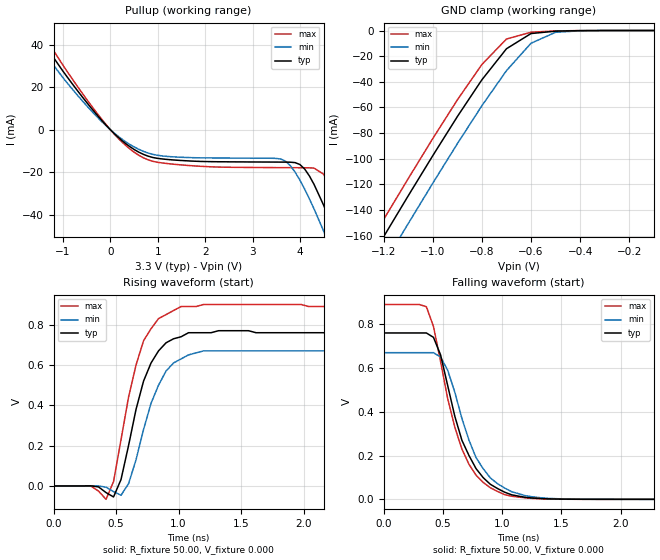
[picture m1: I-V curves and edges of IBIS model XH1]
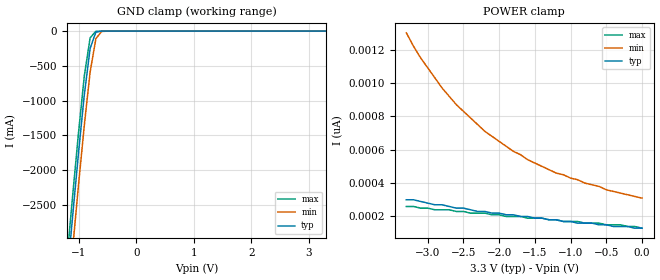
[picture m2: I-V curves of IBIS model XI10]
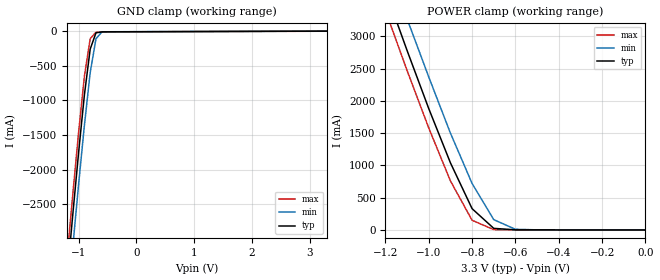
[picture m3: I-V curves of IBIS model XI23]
|   * 9db433a.ibs * IBIS 2.1 Model file
| Rev History
| Rev No.   Description
| 1.0   Initial release   June 6, 2010  lp
[IBIS Ver]   2.1
[Comment char]  |_char
[File name]   9db436a.ibs
[Date]   March 21, 2019
[File Rev]   1.1
[Source]   Originated at Integrated Circuit Systems, Inc.
[Disclaimer] (C) Copyright Integrated Circuit Systems, Inc. 2004
   All rights reserved
ICS hereby grants the user of this IBIS model a non-exclusive,
nontransferable license to use this IBIS model under the following terms.
Before using this IBIS model, the user should read this license.
If the user does not accept these terms,  the IBIS model should be
returned to ICS within 30 days.
   The user is granted this license only to use the IBIS model and
is not granted rights to sell, load, rent, lease or license the IBIS
model in whole or in part, or in modified form to anyone other than
user. User may modify the IBIS model to suit its specific
applications but rights to derivative works and such modifications
shall belong to ICS.
   This IBIS model is provided on an "AS IS" basis and ICS makes
absolutely no warranty with respect to the information contained
herein. ICS DISCLAIMS AND CUSTOMER WAIVES ALL WARRANTIES, EXPRESS
OR IMPLIED, INCLUDING WARRANTIES OF MERCHANTABILITY OR FITNESS FOR
A PARTICULAR PURPOSE. The entire risk as to quality and performance
is with the Customer. ACCORDINGLY, IN NO EVENT SHALL THE COMPANY BE
LIABLE FOR ANY DAMAGES, WHETHER IN CONTRACT OR TORT,INCLUDING ANY
LOST PROFITS OR OTHER INCIDENTAL, CONSEQUENTIAL, EXEMPLARY, OR
PUNITIVE DAMAGES ARISING OUT OF THE USE OR APPLICATION OF THE IBIS
model provided in this package. Further, ICS reserves the right to
make changes without notice to any product herein to improve
reliability, function, or design. ICS does not convey any license
under patent rights or any other intellectual property rights,
including those of third parties.
   ICS is not obligated to provide maintenance or support
for the licensed IBIS model.
|   COMPONENT: ICS9db436a
[Component]   ICS9db436a
[Manufacturer]  ICS
[Package]
| variable   typ   min   max
R_pkg   81.1m   62.2m   100.0m
L_pkg   6.7nH   4.9nH   8.5nH
C_pkg   0.53pF  0.21pF  0.85pF
[Pin]   signal_name   model_name   R_pin   L_pin   C_pin
  1   VDD   POWER   90.5m   4.72nH  0.585pF
  2   SRC_IN   XI4   91.3m   4.11nH  0.57pF
  3   SRC_IN#   XI4   93.6m   3.68nH  0.433pF
  4   GND   GND   39.9m   2.61nH  0.44pF
  5   VDD   POWER   92.1m   3.14nH  0.318pF
  6   DIF_1   XH1   78m   2.79nH  0.286pF
  7   DIF_1#   XH1   70.5m   2.62nH  0.272pF
  8   OE_1(OE_1#)   XI23   39.8m   2.27nH  0.311pF
  9   DIF_2   XH1   74.7m   2.7nH   0.279pF
 10   DIF_2#   XH1   86m   3nH   0.294pF
 11   VDD   POWER   53.2m   2.8nH   0.356pF
 12   BYPASS#/BW   XI23   97.1m   3.84nH  0.432pF
 13   SCLK   XI10   93.6m   4.23nH  0.58pF
 14   SDATA   XIO3   91.4m   4.77nH  0.595pF
 15   GND   GND   91.2m   4.76nH  0.592pF
 16   VDD   POWER   93.7m   4.22nH  0.579pF
 17   SMB_ADR   XI23   97.8m   3.84nH  0.434pF
 18   VDD   POWER   95.6m   3.34nH  0.295pF
 19   DIF_5#   XH1   82.6m   2.93nH  0.285pF
 20   DIF_5   XH1   73.4m   2.67nH  0.277pF
 21   OE_6(OE_6#)   XI23   40m   2.26nH  0.308pF
 22   DIF_6#   XH1   70.8m   2.62nH  0.273pF
 23   DIF_6   XH1   80.8m   2.86nH  0.293pF
 24   VDD   POWER   52.4m   2.73nH  0.378pF
 25   PD#   XI29   40.3m   2.63nH  0.436pF
 26   IREF   XI24   95.1m   3.75nH  0.434pF
 27   GNDA   GND   56.9m   3.8nH   0.63pF
 28   VDDA   POWER   58m   4.46nH  0.642pF
|* Either 3.3V or 2.5V
|** All model are simulated with typical corner process
[Diff Pin]   inv_pin   vdiff   tdelay_typ
2   3   NA   NA
6   7   NA   NA
9   10   NA   NA
20   19   NA   NA
23   22   NA   NA
| Models and submodels in the file (7): XH1 (Open_source), XI10 (Input), XI23 (Input), XI24 (Input), XI29 (Input), XI4 (Input), XIO3 (I/O_open_drain)
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|   Model XH1
[Model]   XH1
Model_type   Open_source
Polarity   Inverting
Vmeas = 0.35V
Cref =   2.00pF
Rref =  500
Vref =   0.0V
C_comp   3.40pF   2.85pF   3.95pF
[Temperature Range]   25.00   70.00   0.000
[Voltage Range]   3.30V   3.00V   3.70V
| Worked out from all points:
|   slope of the pullup table from 0 to 0.495 V, typ, clamps not added: 53.7 ohm
|   GND clamp passes 1 mA (typ) near -0.53 V on its own axis
|   rising waveform, R_fixture 50.00, V_fixture 0.000: 20-80 % time 196ps typ, 209ps min, 191ps max; typ from 0 V to 0.76 V
|   falling waveform, R_fixture 50.00, V_fixture 0.000: 20-80 % time 266ps typ, 276ps min, 255ps max; typ from 0.76 V to 0 V
[Pullup]
| voltage   I(typ)   I(min)   I(max)
-3.3V     120mA      110mA      120mA
-1.9V     57.97mA    52.49mA    62.98mA
-1.5V     43.73mA    39.31mA    47.78mA
-100mV    2.37mA     2.07mA     2.66mA
700mV     -11.65mA   -10.21mA   -13.27mA
3.6V      -15.27mA   -13.83mA   -17.88mA
4V        -16.4mA    -23.77mA   -17.93mA
4.3V      -25.83mA   -37.4mA    -18.11mA
4.5V      -35.53mA   -47.74mA   -20.97mA
4.7V      -46.5mA    -58.63mA   -28.65mA
5.1V      -70.24mA   -81.19mA   -50.61mA
6.6V      -160mA     -170mA     -150mA
[Ramp]
| variable   typ   min   max
dV/dt_r   0.46/0.20n   0.40/0.21n   0.53/0.19n
dV/dt_f   0.45/0.26n   0.40/0.27n   0.53/0.25n
R_load = 50.00
[Rising Waveform]
R_fixture = 50.00
V_fixture = 0.000
V_fixture_min = 0.000
V_fixture_max = 0.000
| time   V(typ)   V(min)   V(max)
0s        -370nV     -380nV     -340nV
300ps     550uV      230uV      -1.44mV
420ps     -32.86mV   -6.35mV    -66.34mV
480ps     -54.44mV   -28.27mV   21.55mV
540ps     32.24mV    -46.01mV   230mV
600ps     200mV      10.91mV    440mV
720ps     520mV      280mV      720mV
840ps     670mV      500mV      830mV
1.02ns    740mV      630mV      890mV
3ns       760mV      670mV      890mV
[Falling Waveform]
R_fixture = 50.00
V_fixture = 0.000
V_fixture_min = 0.000
V_fixture_max = 0.000
| time   V(typ)   V(min)   V(max)
0s        760mV      670mV      890mV
360ps     760mV      670mV      880mV
420ps     740mV      670mV      790mV
480ps     660mV      650mV      630mV
540ps     520mV      590mV      460mV
660ps     270mV      370mV      230mV
780ps     140mV      190mV      110mV
900ps     68.75mV    97.98mV    52.94mV
1.38ns    2.27mV     4.59mV     1.49mV
3ns       -13.74uV   -37.6uV    -15.05uV
[GND_clamp]
| voltage   I(typ)   I(min)   I(max)
-3.3V     -857mA     -877.7mA   -844.3mA
-1.3V     -193.1mA   -214.7mA   -179.6mA
-1.2V     -160.8mA   -182.5mA   -147.3mA
-1.1V     -128.9mA   -150.6mA   -115.5mA
-1V       -97.6mA    -119.1mA   -84.25mA
-900mV    -67.14mA   -88.3mA    -54.11mA
-800mV    -38.43mA   -58.65mA   -26.49mA
-700mV    -14.23mA   -31.32mA   -6.64mA
-600mV    -2.36mA    -9.93mA    -1.32mA
-500mV    -489.3uA   -1.38mA    -326.7uA
-400mV    -91.06uA   -228.9uA   -44.42uA
-100mV    -574.5pA   -10.15nA   -135.8pA
|   Model XI10
[Model]   XI10
Model_type   Input
Polarity   Inverting
Vinl =   0.80V
Vinh =   2.00V
C_comp   3.40pF   2.85pF   3.95pF
[Temperature Range]   27.00   70.00   0.000
[Voltage Range]   3.30V   3.00V   3.70V
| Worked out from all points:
|   GND clamp passes 1 mA (typ) near -0.60 V on its own axis
[GND_clamp]
| voltage   I(typ)   I(min)   I(max)
-3.3V     -24.05A    -24.49A    -23.79A
-1.2V     -3.55A     -4.02A     -3.26A
-1.1V     -2.63A     -3.1A      -2.34A
-1V       -1.74A     -2.2A      -1.45A
-900mV    -910mA     -1.35A     -640mA
-800mV    -250mA     -590mA     -96.82mA
-700mV    -14.58mA   -110mA     -3.87mA
-600mV    -880uA     -5.84mA    -450uA
-500mV    -88.5uA    -350uA     -45.09uA
3.3V      130pA      340pA      120pA
[POWER_clamp]
| voltage   I(typ)   I(min)   I(max)
-3.3V     300pA      1.3nA      260pA
-3.1V     290pA      1.15nA     250pA
-2.9V     270pA      1.03nA     240pA
-2.8V     270pA      970pA      240pA
-2.6V     250pA      870pA      230pA
-2.2V     230pA      710pA      220pA
-1.8V     210pA      590pA      200pA
-1.2V     180pA      460pA      180pA
-900mV    160pA      420pA      170pA
-500mV    150pA      360pA      150pA
-300mV    140pA      340pA      150pA
0V        130pA      310pA      130pA
|   Model XI23
[Model]   XI23
Model_type   Input
Polarity   Inverting
Enable   Active-High
Vinl =   0.80V
Vinh =   2.00V
C_comp   3.40pF   2.85pF   3.95pF
[Temperature Range]   27.00   70.00   0.000
[Voltage Range]   3.30V   3.00V   3.70V
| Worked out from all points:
|   POWER clamp passes 1 mA (typ) near -0.39 V on its own axis
[GND_clamp]
| voltage   I(typ)   I(min)   I(max)
-3.3V     -24.07A    -24.5A     -23.8A
-1.2V     -3.56A     -4.03A     -3.27A
-1.1V     -2.64A     -3.11A     -2.35A
-1V       -1.75A     -2.21A     -1.46A
-900mV    -920mA     -1.36A     -650mA
-800mV    -260mA     -600mA     -110mA
-700mV    -24.92mA   -110mA     -15.24mA
-600mV    -10.96mA   -15.13mA   -11.57mA
-500mV    -9.91mA    -9.4mA     -10.9mA
3.3V      130pA      780uA      -1.03mA
[POWER_clamp]
| voltage   I(typ)   I(min)   I(max)
-3.3V     24.22A     24.67A     23.94A
-1.2V     3.71A      4.2A       3.4A
-1.1V     2.78A      3.27A      2.47A
-1V       1.88A      2.37A      1.58A
-900mV    1.04A      1.5A       760mA
-800mV    330mA      720mA      150mA
-700mV    24.76mA    160mA      5.64mA
-600mV    2.11mA     10.91mA    1.62mA
0V        130pA      310pA      130pA
